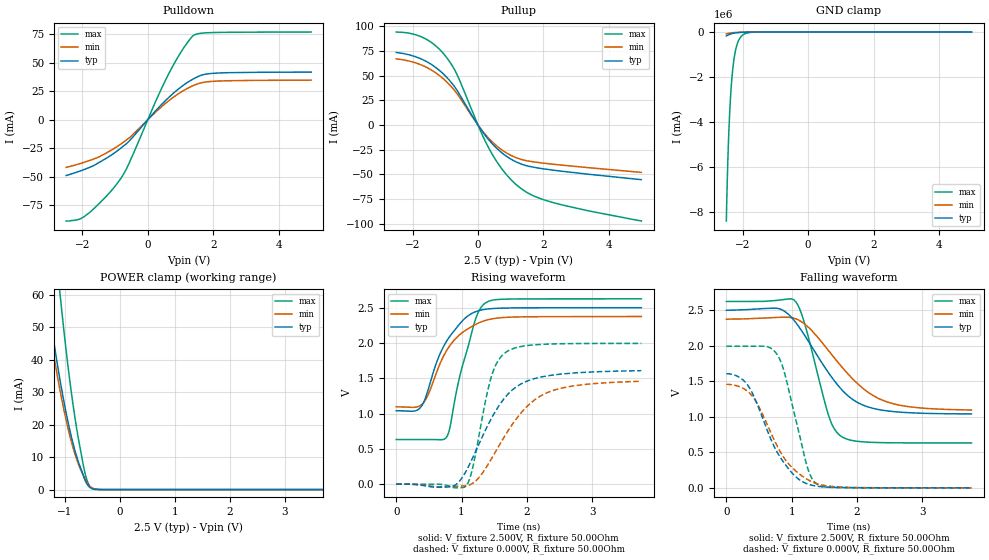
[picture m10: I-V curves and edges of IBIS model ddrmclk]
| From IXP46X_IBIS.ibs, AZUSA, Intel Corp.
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| These Models Have Been correlated to SPICE simulations using the
| JEDEC standard Test Load   p15/n17
[Model]   ddrmclk
Model_type   Output
|Vinl = 900.000mV
|Vinh = 900.000mV
Vmeas = 1.250V
Rref = 50ohm
Cref = 30.000pF
Vref = 1.250V
|   typ   min   max
C_comp   3.000pF   2.700pF   3.300pF
[Voltage Range]   2.500V   2.375V   2.625V
[Temperature Range]   25.0   110.0   -40.0
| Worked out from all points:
|   slope of the pulldown table from 0 to 0.375 V, typ, clamps not added: 31.5 ohm
|   slope of the pullup table from 0 to 0.375 V, typ, clamps not added: 22.4 ohm
|   POWER clamp passes 1 mA (typ) near -0.56 V on its own axis
|   falling waveform, V_fixture 2.500V, R_fixture 50.00Ohm: 20-80 % time 663ps typ, 760ps min, 336ps max; typ from 2.5 V to 1.04 V
|   rising waveform, V_fixture 2.500V, R_fixture 50.00Ohm: 20-80 % time 430ps typ, 448ps min, 312ps max; typ from 1.04 V to 2.5 V
|   rising waveform, V_fixture 0.000V, R_fixture 50.00Ohm: 20-80 % time 578ps typ, 667ps min, 274ps max; typ from 0 V to 1.61 V
|   falling waveform, V_fixture 0.000V, R_fixture 50.00Ohm: 20-80 % time 485ps typ, 515ps min, 311ps max; typ from 1.61 V to 0 V
[Pulldown]
|   Voltage   I(typ)   I(min)   I(max)
-2.5V     -49.09mA   -41.96mA   -89mA
-2.115V   -45.56mA   -38.98mA   -87.59mA
-1.855V   -42.78mA   -36.62mA   -83.16mA
-1.275V   -33.99mA   -29.38mA   -67.4mA
-865mV    -25.95mA   -22.23mA   -53.25mA
-605mV    -19.86mA   -16.86mA   -40.25mA
595mV     18.25mA    15.52mA    37.76mA
995mV     28.2mA     23.81mA    58.45mA
1.395V    35.78mA    29.94mA    73.85mA
1.66V     39.18mA    32.48mA    75.9mA
2.13V     40.84mA    33.81mA    76.49mA
4.995V    41.7mA     34.63mA    76.85mA
[GND Clamp]
|   Voltage   I(typ)   I(min)   I(max)
-2.5V     -174.7A    -83.13A    -8.409kA
-2.485V   -161A      -77.27A    -7.418kA
-2.465V   -144.5A    -70.14A    -6.284kA
-2.425V   -116.3A    -57.81A    -4.51kA
-2.38V    -91.22A    -46.52A    -3.105kA
-2.325V   -67.79A    -35.68A    -1.968kA
-2.265V   -49.06A    -26.74A    -1.198kA
-2.195V   -33.68A    -19.11A    -670.9A
-2.11V    -21.36A    -12.74A    -332.3A
-2V       -11.88A    -7.554A    -134.1A
-1.5V     -878.7mA   -738.2mA   -2.334A
4.995V    0A         0A         0A
[Pullup]
|   Voltage   I(typ)   I(min)   I(max)
-2.5V     73.44mA    66.97mA    94.14mA
-1.705V   66.41mA    60.42mA    88.91mA
-1.375V   60.2mA     54.67mA    82.39mA
-1.01V    50.09mA    45.35mA    70.48mA
-645mV    35.32mA    32mA       51.36mA
75mV      -3.774mA   -3.418mA   -5.849mA
395mV     -17.48mA   -15.76mA   -27.29mA
825mV     -30.59mA   -27.35mA   -48.49mA
1.295V    -39.19mA   -34.6mA    -63.79mA
1.72V     -42.9mA    -37.43mA   -72.11mA
2.34V     -45.93mA   -39.88mA   -78.96mA
4.995V    -55.38mA   -48mA      -97.25mA
[POWER Clamp]
|   Voltage   I(typ)   I(min)   I(max)
-2.5V     256.4mA    235.2mA    408.3mA
-1.415V   71.99mA    65.47mA    123.8mA
-1.355V   64.16mA    58.31mA    111mA
-1.315V   59.14mA    53.72mA    102.8mA
-1.095V   34.54mA    31.31mA    61.62mA
-1.065V   31.62mA    28.65mA    56.64mA
-930mV    19.91mA    18.05mA    36.32mA
-770mV    9.398mA    8.607mA    17.32mA
-635mV    2.984mA    3.527mA    5.21mA
-575mV    1.204mA    1.652mA    1.901mA
-515mV    392.7uA    639.4uA    431.7uA
4.995V    0A         0A         0A
[Ramp]
R_load = 50.00Ohm
|   typ   min   max
dV/dt_r   964.672mV/577.567ps 875.052mV/666.393ps   1.196V/273.717ps
dV/dt_f   875.701mV/663.089ps 767.445mV/759.584ps   1.196V/335.711ps
[Falling Waveform]
V_fixture = 2.500V
V_fixture_min = 2.375V
V_fixture_max = 2.625V
R_fixture = 50.00Ohm
|   Time   V(typ)   V(min)   V(max)
0s        2.5V       2.375V     2.625V
780ps     2.528V     2.4V       2.641V
1.06ns    2.331V     2.381V     2.623V
1.2ns     2.144V     2.305V     2.306V
1.58ns    1.599V     1.914V     976.4mV
1.67ns    1.487V     1.81V      805.4mV
1.78ns    1.368V     1.688V     712.8mV
2.06ns    1.178V     1.424V     650.3mV
2.46ns    1.084V     1.21V      635.4mV
3.75ns    1.04V      1.096V     632mV
[Rising Waveform]
V_fixture = 2.500V
V_fixture_min = 2.375V
V_fixture_max = 2.625V
R_fixture = 50.00Ohm
|   Time   V(typ)   V(min)   V(max)
0s        1.04V      1.096V     632mV
380ps     1.096V     1.12V      632mV
490ps     1.343V     1.27V      632.2mV
630ps     1.755V     1.615V     630.8mV
770ps     2.024V     1.891V     666.9mV
820ps     2.094V     1.962V     795.7mV
980ps     2.28V      2.124V     1.558V
1.19ns    2.434V     2.25V      2.268V
1.38ns    2.48V      2.324V     2.576V
3.75ns    2.5V       2.375V     2.625V
[Rising Waveform]
V_fixture = 0.000V
V_fixture_min = 0.000V
V_fixture_max = 0.000V
R_fixture = 50.00Ohm
|   Time   V(typ)   V(min)   V(max)
0s        362.4nV    1.8uV      -7.065nV
840ps     -33.81mV   -33.59mV   -36.89mV
1.07ns    186.8mV    -21.74mV   -23.25mV
1.17ns    374.1mV    12.04mV    233.1mV
1.46ns    937.6mV    365mV      1.536V
1.57ns    1.108V     541.4mV    1.764V
1.71ns    1.276V     755.6mV    1.887V
2.02ns    1.467V     1.118V     1.965V
2.35ns    1.54V      1.311V     1.985V
3.75ns    1.608V     1.458V     1.994V
[Falling Waveform]
V_fixture = 0.000V
V_fixture_min = 0.000V
V_fixture_max = 0.000V
R_fixture = 50.00Ohm
|   Time   V(typ)   V(min)   V(max)
0s        1.608V     1.458V     1.994V
180ps     1.567V     1.431V     1.994V
350ps     1.415V     1.34V      1.994V
640ps     777.8mV    861.1mV    1.984V
780ps     497.8mV    585mV      1.874V
900ps     331.1mV    399.8mV    1.585V
1.24ns    55.45mV    117.8mV    289.8mV
1.31ns    36.62mV    84.87mV    130.8mV
1.4ns     21.96mV    54.58mV    43.79mV
3.75ns    362.4nV    1.8uV      -7.065nV
